(* 	
	Program Name: 	ACS_MOVE_HOME
	Purpose:		Copy Home Move Profile to ACS Drive Output Registers
	When Executed:	Primes Output Registers for an Home Move to be executed upon Start Motion command
*)
PROGRAM ACS_MOVE_HOME
VAR_IN_OUT
	Axis:ACS_DRIVE_TYPE;
END_VAR

VAR_INPUT

END_VAR

VAR
	_moveType:UDINT := ACS_MOTION_TYPES.HOME;
	// Target Index
	_moveSelect:USINT := 0;
END_VAR

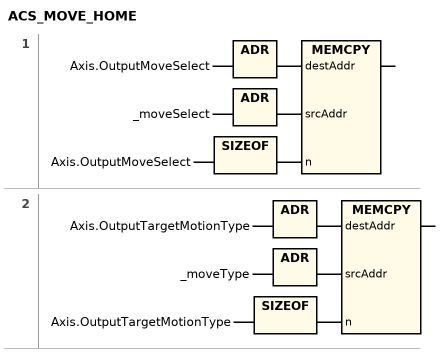
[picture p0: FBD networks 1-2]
// NETWORK 1
MEMCPY(destAddr := ADR(Axis.OutputMoveSelect), srcAddr := ADR(_moveSelect), n := SIZEOF(Axis.OutputMoveSelect));

// NETWORK 2
MEMCPY(destAddr := ADR(Axis.OutputTargetMotionType), srcAddr := ADR(_moveType), n := SIZEOF(Axis.OutputTargetMotionType));

END_PROGRAM
